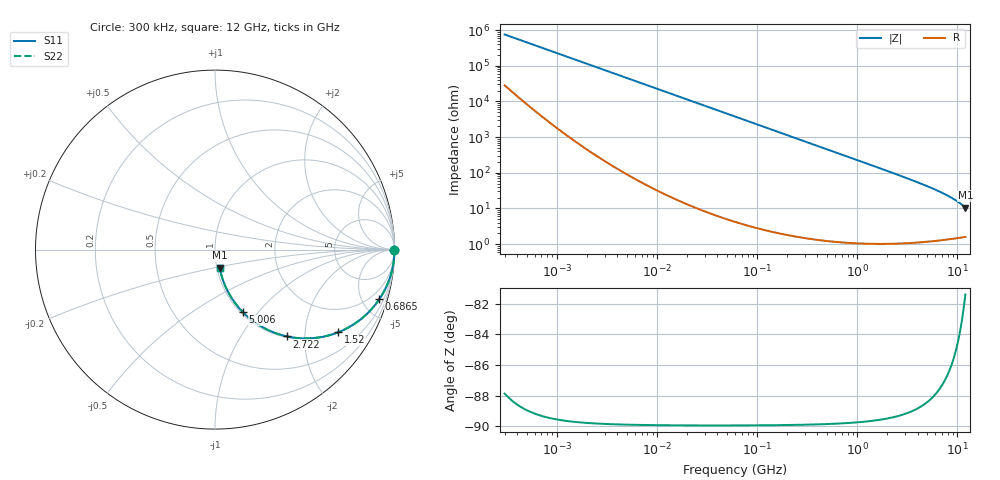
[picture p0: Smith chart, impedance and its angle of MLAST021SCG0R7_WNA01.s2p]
! MLAST021SCG0R7_WNA01  S-PARAMETER MODEL  ( General Type )
! Model Generated by TAIYO YUDEN Corporation (http://www.ty-top.com)
! Version 1.0
! TAIYO YUDEN Control No. 220901
! Copyright(c) 2022 TAIYO YUDEN CO.,LTD. All Rights Reserved.
! Product Description (link to TY-COMPAS)
! https://ds.yuden.co.jp/TYCOMPAS/or/detail?pn=MLAST021SCG0R7BWNA01&u=M
! Products Name : Multilayer Ceramic Capacitors
! Characteristics :
!  Capacitance : 0.7 pF , Rated Voltage : 25V , TCC : CG / C0G
!  Case Size : 0.25 x 0.125 / 0.0098 x 0.0049 [mm/inch] , Thickness : 0.125 / 0.0049 [mm/inch]
!  (Conditions: Temperature = 25 degC , DC Bias Current/Voltage = 0A / 0V)
! External Node Assignments :
!  1  o---| |---o  2
! GND o---------o GND
! Frequency Range : 0.3MHz  -  12000MHz  [ 401 STEP ]
# MHz S RI R 50
! Freq[MHz].  S11 Real  S11 Imag  S21 Real  S21 Imag  S12 Real  S12 Imag  S22 Real  S22 Imag
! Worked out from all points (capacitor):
!   401 points, 300 kHz to 12 GHz, reference 50 ohm
!   read as one part in series: C = 700 fF near 316.3 kHz
!   lowest |Z| = 10.6 ohm at 12 GHz (marker M1)
!   S11 on the Smith chart (normalised r, x): 300 kHz: open; 686.5 MHz: 1.02, -6.61; 1.52 GHz: 1.02, -2.97; 2.722 GHz: 1.02, -1.63; 5.006 GHz: 1.02, -0.84; 12 GHz: 1.03, -0.21
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0.3  1 -0.000132  4.93e-06 0.000132  4.93e-06 0.000132  1 -0.000132
0.316324  1 -0.000139  4.85e-06 0.000139  4.85e-06 0.000139  1 -0.000139
1.769972  1 -0.000778  4.02e-06 0.000778  4.02e-06 0.000778  1 -0.000778
10.44266  1 -0.00459  2.74e-05 0.00459  2.74e-05 0.00459  1 -0.00459
60  0.9993 -0.0264  0.000725 0.0264  0.000725 0.0264  0.9993 -0.0264
164.1901  0.9947 -0.0718  0.00529 0.0718  0.00529 0.0718  0.9947 -0.0718
244.3004  0.9884 -0.1062  0.0116 0.1062  0.0116 0.1062  0.9884 -0.1062
353.9943  0.976 -0.152  0.024 0.152  0.024 0.152  0.976 -0.152
512.9422  0.951 -0.2146  0.049 0.2146  0.049 0.2146  0.951 -0.2146
686.4755  0.9155 -0.2765  0.0845 0.2765  0.0845 0.2765  0.9155 -0.2765
1021.415  0.83 -0.3733  0.17 0.3733  0.17 0.3733  0.83 -0.3733
1229.528  0.7708 -0.4175  0.2292 0.4175  0.2292 0.4175  0.7708 -0.4175
1519.776  0.6869 -0.4603  0.3131 0.4603  0.3131 0.4603  0.6869 -0.4603
2088.533  0.5353 -0.494  0.4647 0.494  0.4647 0.494  0.5353 -0.494
2722.03  0.401 -0.4838  0.599 0.4838  0.599 0.4838  0.401 -0.4838
3740.715  0.2567 -0.4275  0.7433 0.4275  0.7433 0.4275  0.2567 -0.4275
5006.236  0.1561 -0.3494  0.8439 0.3494  0.8439 0.3494  0.1561 -0.3494
6524.734  0.0933 -0.2708  0.9067 0.2708  0.9067 0.2708  0.0933 -0.2708
8064.993  0.0597 -0.2088  0.9403 0.2088  0.9403 0.2088  0.0597 -0.2088
9708.23  0.04 -0.1568  0.96 0.1568  0.96 0.1568  0.04 -0.1568
11380.75  0.0288 -0.1143  0.9712 0.1143  0.9712 0.1143  0.0288 -0.1143
12000  0.026 -0.1005  0.974 0.1005  0.974 0.1005  0.026 -0.1005
